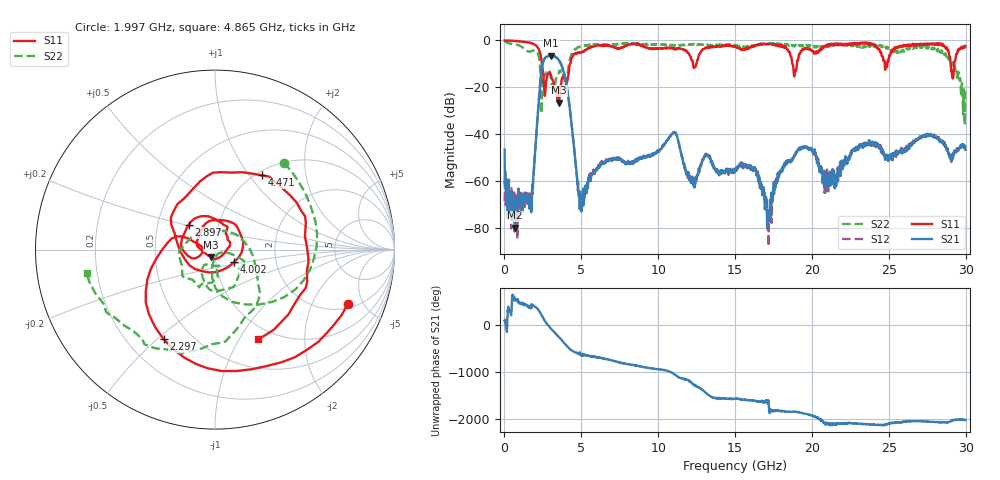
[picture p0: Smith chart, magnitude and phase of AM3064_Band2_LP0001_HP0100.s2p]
# Hz S DB R 50.0
!freq dBS11 angS11 dBS21 angS21 dBS12 angS12 dBS22 angS22
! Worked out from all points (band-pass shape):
!   1600 points, 10 MHz to 29.98 GHz, reference 50 ohm
!   highest |S21| = -6.47 dB at 3.046 GHz (marker M1); lowest = -79.7 dB at 684.8 MHz (marker M2)
!   |S21| within 3 dB of the highest: 2.507 GHz to 3.638 GHz (1.131 GHz wide, 36.8 % of centre)
!   lowest |S11| = -26.4 dB at 3.553 GHz (marker M3), VSWR 1.10, Z = 47.7 - j4.05 ohm
!   |S11| at or under -10 dB: 2.436 GHz to 4.268 GHz (1.832 GHz wide, 54.6 % of centre); 12.26 GHz to 12.48 GHz (218.9 MHz wide, 1.77 % of centre); 18.73 GHz to 19.02 GHz (291.3 MHz wide, 1.54 % of centre)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
!   |S22| runs from -36.0 to -0.2 dB; largest |S21 - S12| = 0.015
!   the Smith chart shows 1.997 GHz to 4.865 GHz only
!   S11 on the Smith chart (normalised r, x): 1.997 GHz: 2.28, -3.82; 2.297 GHz: 0.35, -0.52; 2.897 GHz: 0.72, +0.20; 4.002 GHz: 1.22, -0.18; 4.471 GHz: 1.06, +1.15; 4.865 GHz: 0.84, -1.21
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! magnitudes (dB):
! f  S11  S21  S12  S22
! 10 MHz  0.0  -46.4  -68.4  -0.2
! 684.8 MHz  -0.2  -79.7  -74.1  -1.7
! 1.697 GHz  -1.1  -70.3  -67.1  -4.7
! 1.997 GHz  -1.9  -47.1  -46.8  -4.2
! 2.297 GHz  -4.8  -20.0  -20.0  -10.2
! 2.897 GHz  -13.9  -6.7  -6.6  -12.6
! 3.046 GHz  -15.4  -6.5  -6.5  -17.1
! 3.553 GHz  -26.4  -8.7  -8.5  -13.2
! 4.002 GHz  -18.0  -17.6  -17.7  -18.6
! 4.471 GHz  -6.2  -42.5  -42.1  -4.4
! 4.865 GHz  -5.1  -66.5  -65.4  -2.8
! 5.015 GHz  -5.1  -72.8  -66.8  -2.6
! 10 GHz  -3.5  -46.8  -47.3  -1.8
! 15 GHz  -2.6  -55.3  -55.8  -1.9
! 16.34 GHz  -2.3  -54.8  -56.2  -2.2
! 17.24 GHz  -1.4  -75.2  -75.9  -1.3
! 18.19 GHz  -2.4  -53.1  -52.9  -1.9
! 19.99 GHz  -4.1  -46.9  -46.1  -2.1
! 20.8 GHz  -2.5  -58.2  -55.9  -2.6
! 25 GHz  -8.2  -49.4  -50.2  -3.0
! 28.56 GHz  -2.1  -44.0  -43.3  -5.0
! 29.98 GHz  -2.3  -46.6  -46.0  -21.7
